FUNCTION_BLOCK FileExample01_Gcode	//3x3 flyways 1 xbot - DeleteGCode,SaveGCode,ReadGCode,GetGCodeIDs,RunGCode. G-code file 'GCodeDemo.txt' must be on disc in the DemoFilesFolder.  
VAR_INPUT
	Execute : BOOL;
	DemoFilesFolder : STRING(255);	//Folder that contains the GCodeDemo.txt file
END_VAR
VAR_OUTPUT
	Done : BOOL;
END_VAR
VAR_IN_OUT
	PM_Controller : PMControllerType;	// the planar motor controller to use
END_VAR
VAR
	Read_file : ReadFileOnDisk;
	sent_Gcode_data : ARRAY[0..199999] OF SINT;
	sent_data_size : DINT;
	PMC_DeleteGCode1 : PMC_GCode_DeleteGCode;
	PMC_SaveGCode1 : PMC_GCode_SaveGCode;
	PMC_ReadGCode1 : PMC_GCode_ReadGCode;
	read_Gcode_data : ARRAY[0..199999] OF SINT;	
	read_data_size : DINT;
	PMC_GetGCodeIDs : PMC_GCode_GetGCodeIDs;
	PMC_RunGCode1 : PMC_GCode_RunGCode;
END_VAR

//3x3 flyways 1 xbot - DeleteGCode,SaveGCode,ReadGCode,GetGCodeIDs,RunGCode. G-code file 'GCodeDemo.txt' must be on disc in the DemoFilesFolder.  

//Read testing G-code file from disk 
Read_file(Execute := Execute,file_path := CONCAT(STR1 := DemoFilesFolder,STR2 := '\GCodeDemo.txt'),buffer_size := 200000,file_size => sent_data_size,data := sent_Gcode_data);

//Delete G-code file ID 1
PMC_DeleteGCode1(Execute := Read_file.Done,GCodeID := 1,PM_Controller := PM_Controller);

//Send the testing G-code file to the PMC
PMC_SaveGCode1(Execute := PMC_DeleteGCode1.Done,GCodeID := 1,nBytes := sent_data_size,Bytes := sent_Gcode_data,PM_Controller := PM_Controller);

//Read back the G-code file from the PMC
PMC_ReadGCode1(Execute := PMC_SaveGCode1.Done,GCodeID := 1,nBytes => read_data_size,Bytes := read_Gcode_data,PM_Controller := PM_Controller);

//Get the IDs of the G-code files on the PMC
PMC_GetGCodeIDs(Execute := PMC_ReadGCode1.Done,PM_Controller := PM_Controller);

//Run the testing G-code file
PMC_RunGCode1(Execute := PMC_GetGCodeIDs.Done,cmdLB := 3,GCodeID := 1,XbotID := 1,PM_Controller := PM_Controller);

Done := PMC_RunGCode1.Done;

END_FUNCTION_BLOCK
